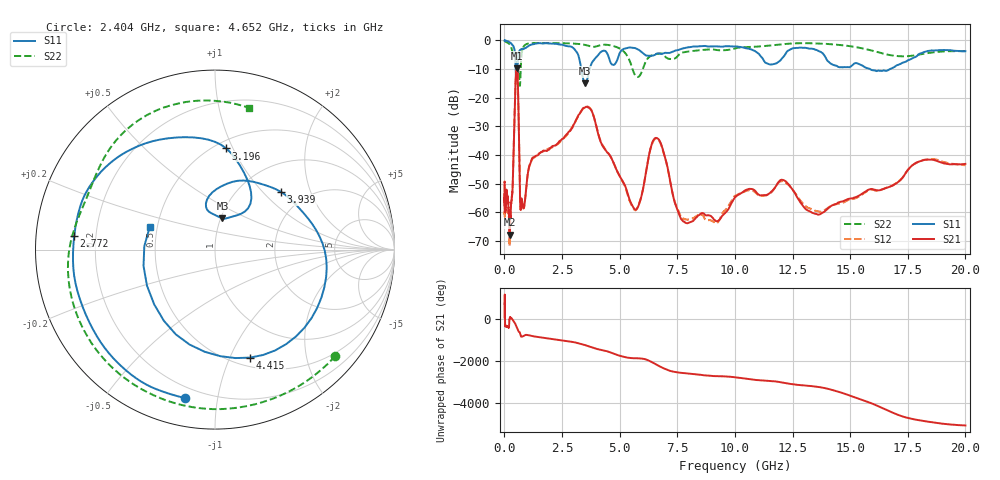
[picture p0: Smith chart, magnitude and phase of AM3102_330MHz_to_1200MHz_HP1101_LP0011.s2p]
! Date/Time: Tue, Sep 11, 2018 5:22 PM
! Network Analyzer: Agilent Technologies E8362B Rev: A.07.50.63
! Sweep from 0.010 to 20.000 GHz, 1601 Points, Sweep Type: LOG
! Power Supply: 4.949 V, 0.001 A
# Hz S DB R 50
!freq MagS11 AngS11 MagS21 AngS21 MagS12 AngS12 MagS22 AngS22
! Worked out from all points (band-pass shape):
!   1601 points, 10 MHz to 20 GHz, reference 50 ohm
!   highest |S21| = -9.68 dB at 538.2 MHz (marker M1); lowest = -67.8 dB at 234.4 MHz (marker M2)
!   |S21| within 3 dB of the highest: 494.6 MHz to 573.7 MHz (79.16 MHz wide, 14.8 % of centre)
!   lowest |S11| = -15.0 dB at 3.498 GHz (marker M3), VSWR 1.43, Z = 51.1 + j18.3 ohm
!   |S11| at or under -10 dB: 486.6 MHz to 561.4 MHz (74.72 MHz wide, 14.3 % of centre); 3.34 GHz to 3.7 GHz (360.1 MHz wide, 10.2 % of centre); 15.86 GHz to 16.74 GHz (877.6 MHz wide, 5.38 % of centre)
!   |S22| runs from -15.8 to -0.2 dB; largest |S21 - S12| = 0.0065
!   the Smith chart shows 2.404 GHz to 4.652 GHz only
!   S11 on the Smith chart (normalised r, x): 2.404 GHz: 0.14, -0.81; 2.772 GHz: 0.12, +0.05; 3.196 GHz: 0.57, +0.94; 3.939 GHz: 1.51, +1.28; 4.415 GHz: 0.59, -1.19; 4.652 GHz: 0.45, +0.13
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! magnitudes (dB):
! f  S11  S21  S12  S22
! 10 MHz  0.0  -49.4  -50.6  -0.2
! 35.55 MHz  -0.1  -58.5  -57.7  -0.3
! 126.4 MHz  -0.2  -54.5  -55.2  -0.8
! 234.4 MHz  -0.7  -67.8  -69.0  -1.4
! 356 MHz  -1.7  -51.3  -51.6  -4.4
! 447.2 MHz  -3.6  -24.2  -24.2  -4.1
! 538.2 MHz  -12.0  -9.7  -9.7  -10.8
! 594.7 MHz  -6.2  -17.9  -18.0  -11.2
! 702.3 MHz  -3.3  -59.0  -58.8  -11.7
! 1.59 GHz  -1.0  -39.0  -39.0  -0.9
! 2.404 GHz  -1.5  -35.0  -35.5  -1.0
! 2.772 GHz  -2.1  -32.1  -32.4  -1.0
! 3.196 GHz  -4.9  -26.3  -26.4  -1.2
! 3.498 GHz  -15.0  -23.4  -23.3  -1.6
! 3.939 GHz  -6.2  -28.4  -28.4  -2.2
! 4.415 GHz  -4.0  -38.6  -38.4  -1.5
! 4.652 GHz  -8.3  -41.2  -41.3  -1.8
! 5.652 GHz  -2.7  -58.9  -59.1  -11.9
! 6.58 GHz  -4.8  -34.0  -34.2  -4.8
! 7.958 GHz  -2.4  -63.7  -62.6  -3.9
! 13.68 GHz  -3.9  -60.7  -59.8  -1.1
! 20 GHz  -3.8  -43.1  -43.5  -3.7
